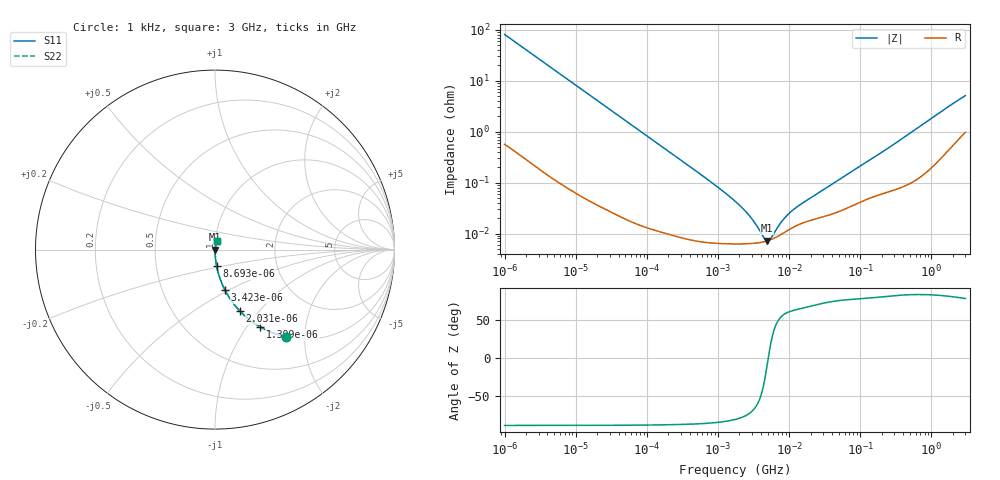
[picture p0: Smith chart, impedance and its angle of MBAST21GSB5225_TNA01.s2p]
! MBAST21GSB5225_TNA01  S-PARAMETER MODEL  ( Standard Model )
! Model Generated by TAIYO YUDEN Corporation (http://www.ty-top.com)
! Version 1.0
! TAIYO YUDEN Control No. 220601
! Copyright(c) 2012 TAIYO YUDEN CO.,LTD. All Rights Reserved.
! Product Description (link to TY-COMPAS)
! https://ds.yuden.co.jp/TYCOMPAS/or/detail?pn=MBAST21GSB5225KTNA01&u=M
! Products Name : Multilayer Ceramic Capacitors
! Characteristics :
!  Capacitance : 2.2 [uF] , Rated Voltage : 25 [V] , TCC : X5R
!  Case Size : 2.0 x 1.25 / 0.079 x 0.049 [mm/inch] , Thickness : 1.25 / 0.049 [mm/inch]
!  (Conditions: Temperature = 25 [degC] , DC Bias Voltage = 0 [V])
! External Node Assignments :
!  1  o---| |---o  2
! GND o---------o GND
! Frequency Range : 1kHz  -  3GHz  [ 401 STEP ]
# MHZ S RI R 50
! Freq[MHz].  S11 Real  S11 Imag  S21 Real  S21 Imag  S12 Real  S12 Imag  S22 Real  S22 Imag
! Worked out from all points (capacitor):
!   401 points, 1 kHz to 3 GHz, reference 50 ohm
!   read as one part in series: C = 1.96 uF near 1.077 kHz
!   lowest |Z| = 7.26 mohm at 4.92 MHz (marker M1)
!   series resonance near 5.085 MHz, so ESL is about 500 pH
!   S11 on the Smith chart (normalised r, x): 1 kHz: 1.01, -1.62; 1.399 kHz: 1.01, -1.16; 2.031 kHz: 1.01, -0.80; 3.423 kHz: 1.00, -0.48; 8.693 kHz: 1.00, -0.19; 3 GHz: 1.02, +0.10
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0.001  0.3968 -0.4858  0.6032 0.4858  0.6032 0.4858  0.3968 -0.4858
0.001399  0.2533 -0.4314  0.7467 0.4314  0.7467 0.4314  0.2533 -0.4314
0.002031  0.1398 -0.3433  0.8602 0.3433  0.8602 0.3433  0.1398 -0.3433
0.003423  0.055 -0.2245  0.945 0.2245  0.945 0.2245  0.055 -0.2245
0.008693  0.00945 -0.0931  0.9906 0.0931  0.9906 0.0931  0.00945 -0.0931
0.01216  0.00503 -0.067  0.995 0.067  0.995 0.067  0.00503 -0.067
0.033275  0.000863 -0.0247  0.9991 0.0247  0.9991 0.0247  0.000863 -0.0247
0.147855  0.000141 -0.0056  0.9999 0.0056  0.9999 0.0056  0.000141 -0.0056
0.762639  6.69e-05 -0.00107  0.9999 0.00107  0.9999 0.00107  6.69e-05 -0.00107
1.732051  6.28e-05 -0.000429  0.9999 0.000429  0.9999 0.000429  6.28e-05 -0.000429
2.709407  6.34e-05 -0.000223  0.9999 0.000223  0.9999 0.000223  6.34e-05 -0.000223
3.93371  6.68e-05 -8.6e-05  0.9999 8.6e-05  0.9999 8.6e-05  6.68e-05 -8.6e-05
4.238263  6.81e-05 -6.06e-05  0.9999 6.06e-05  0.9999 6.06e-05  6.81e-05 -6.06e-05
4.919932  7.18e-05 -1.09e-05  0.9999 1.09e-05  0.9999 1.09e-05  7.18e-05 -1.09e-05
5.711239  7.74e-05 3.82e-05  0.9999 -3.82e-05  0.9999 -3.82e-05  7.74e-05 3.82e-05
6.153411  8.1e-05 6.26e-05  0.9999 -6.26e-05  0.9999 -6.26e-05  8.1e-05 6.26e-05
7.988506  9.89e-05 0.000147  0.9999 -0.000147  0.9999 -0.000147  9.89e-05 0.000147
9.991309  0.000119 0.000219  0.9999 -0.000219  0.9999 -0.000219  0.000119 0.000219
21.06097  0.000186 0.000491  0.9998 -0.000491  0.9998 -0.000491  0.000186 0.000491
256.0921  0.000689 0.00489  0.9993 -0.00489  0.9993 -0.00489  0.000689 0.00489
1591.635  0.00456 0.0282  0.9954 -0.0282  0.9954 -0.0282  0.00456 0.0282
3000  0.0121 0.0491  0.9879 -0.0491  0.9879 -0.0491  0.0121 0.0491
